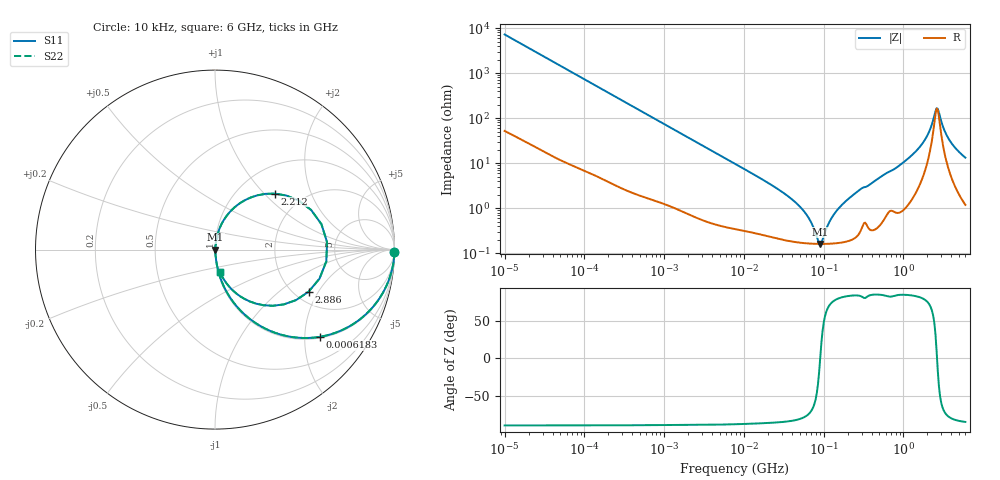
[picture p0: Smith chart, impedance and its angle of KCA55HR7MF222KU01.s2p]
!Murata Part Number: KCA55HR7MF222KU01
!These Parameters are Measured in Series Mode Connection
!Data Generated on Jan 08, 2026
!  o--ll--o
!Port1  Port2
!  o------o
!Operation Temp=25[degC], DC Bias Voltage=0[V]
!Freq. Start=10[kHz] Stop=6[GHz] 401[Steps]
# Hz S RI R 50
!Freq.(Hz) S11(Real) S11(Imag) S21(Real) S21(Imag) S12(Real) S12(Imag) S22(Real) S22(Imag)
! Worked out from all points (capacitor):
!   401 points, 10 kHz to 6 GHz, reference 50 ohm
!   read as one part in series: C = 2.2 nF near 10.69 kHz
!   lowest |Z| = 161 mohm at 90.79 MHz (marker M1)
!   series resonance near 90.63 MHz, so ESL is about 1.4 nH
!   S11 on the Smith chart (normalised r, x): 10 kHz: open; 618.3 kHz: 1.03, -2.39; 2.212 GHz: 1.46, +1.15; 2.886 GHz: 2.37, -1.65; 6 GHz: 1.02, -0.26
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10000  0.9997 -0.0138  0.000292 0.0138  0.000292 0.0138  0.9997 -0.0138
92862  0.9829 -0.125  0.0171 0.125  0.0171 0.125  0.9829 -0.125
269211  0.8788 -0.321  0.1212 0.321  0.1212 0.321  0.8788 -0.321
618339  0.5862 -0.4856  0.4138 0.4856  0.4138 0.4856  0.5862 -0.4856
862344  0.4252 -0.4865  0.5748 0.4865  0.5748 0.4865  0.4252 -0.4865
2188524  0.1092 -0.302  0.8908 0.302  0.8908 0.302  0.1092 -0.302
7745967  0.0126 -0.0953  0.9874 0.0953  0.9874 0.0953  0.0126 -0.0953
3.823436e7  0.00211 -0.0167  0.9979 0.0167  0.9979 0.0167  0.00211 -0.0167
5.512555e7  0.00176 -0.0089  0.9982 0.0089  0.9982 0.0089  0.00176 -0.0089
7.193098e7  0.00164 -0.00402  0.9984 0.00402  0.9984 0.00402  0.00164 -0.00402
9.078908e7  0.0016 3.17e-05  0.9984 -3.17e-05  0.9984 -3.17e-05  0.0016 3.17e-05
1.266156e8  0.00166 0.00591  0.9983 -0.00591  0.9983 -0.00591  0.00166 0.00591
1.708031e8  0.00187 0.0118  0.9981 -0.0118  0.9981 -0.0118  0.00187 0.0118
6.67969e8  0.0124 0.0629  0.9876 -0.0629  0.9876 -0.0629  0.0124 0.0629
1.58612e9  0.0729 0.1982  0.9271 -0.1982  0.9271 -0.1982  0.0729 0.1982
1.936459e9  0.1693 0.2767  0.8307 -0.2767  0.8307 -0.2767  0.1693 0.2767
2.212024e9  0.3346 0.3118  0.6654 -0.3118  0.6654 -0.3118  0.3346 0.3118
2.612262e9  0.6243 0.0416  0.3757 -0.0416  0.3757 -0.0416  0.6243 0.0416
2.886376e9  0.5211 -0.235  0.4789 0.235  0.4789 0.235  0.5211 -0.235
3.189254e9  0.3223 -0.3129  0.6777 0.3129  0.6777 0.3129  0.3223 -0.3129
3.766309e9  0.1406 -0.2603  0.8594 0.2603  0.8594 0.2603  0.1406 -0.2603
6e9  0.0282 -0.1266  0.9718 0.1266  0.9718 0.1266  0.0282 -0.1266
